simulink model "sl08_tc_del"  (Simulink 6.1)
settings: Solver=ode45  StartTime=0.0  StopTime=0.1  MaxStep=0.001  RelTol=1e-3
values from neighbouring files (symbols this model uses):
  G1den = [0.05 15.008 2.4]    [sl08.m]
  G1num = 1.5    [sl08.m]
  G2den = [6.25 1]    [sl08.m]
  G2num = 12.5    [sl08.m]
  Ts = 0.005    [sl08.m]
undefined symbols (not defined in the file or in its folder): Rden, Rnum

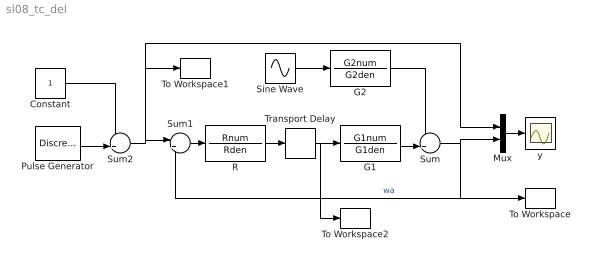
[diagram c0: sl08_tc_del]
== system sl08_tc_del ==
  Constant : Constant  Value=1
  G1 : TransferFcn  Numerator=G1num  Denominator=G1den  AbsoluteTolerance=auto  Realization=auto
  G2 : TransferFcn  Numerator=G2num  Denominator=G2den  AbsoluteTolerance=auto  Realization=auto
  Mux : Mux  Inputs=2
  Pulse Generator : DiscretePulseGenerator  PulseType=Time-based  Amplitude=2  Period=0.2  PulseWidth=50  PhaseDelay=0
  R : TransferFcn  Numerator=Rnum  Denominator=Rden  AbsoluteTolerance=auto  Realization=auto
  Sine Wave : Sin  SineType=Time-based  Amplitude=0  Bias=0  Frequency=50  Phase=0  Samples=10
  Sum : Sum  Inputs=++|  SaturateOnIntegerOverflow=on
  Sum1 : Sum  Inputs=|+-  SaturateOnIntegerOverflow=on
  Sum2 : Sum  Inputs=-+|  SaturateOnIntegerOverflow=on
  To Workspace : ToWorkspace  VariableName=ycd  SaveFormat=Array
  To Workspace1 : ToWorkspace  VariableName=wcd  SaveFormat=Array
  To Workspace2 : ToWorkspace  VariableName=ucd  SaveFormat=Array
  Transport Delay : TransportDelay  DelayTime=Ts/2  InitialInput=0  BufferSize=1024  PadeOrder=0
  y : Scope
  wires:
  R/1 -> Transport Delay/1
  Sum/1 -> Mux/2, Sum1/2, To Workspace/1  "wa"
  Sum1/1 -> R/1
  Sine Wave/1 -> G2/1
  G1/1 -> Sum/2
  G2/1 -> Sum/1
  Sum2/1 -> Sum1/1, Mux/1, To Workspace1/1
  Pulse Generator/1 -> Sum2/2
  Constant/1 -> Sum2/1
  Mux/1 -> y/1
  Transport Delay/1 -> G1/1, To Workspace2/1
